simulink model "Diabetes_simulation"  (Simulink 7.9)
settings: Solver=ode4  SolverMode=SingleTasking  StartTime=0.0  StopTime=2880  FixedStep=parameters.passo_int  RelTol=1e-3
undefined symbols (not defined in the file or in its folder): boluses, meals, parameters
libraries: simulink x1

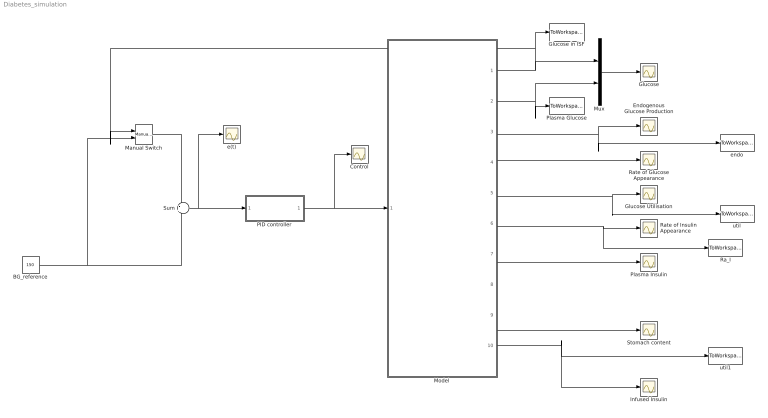
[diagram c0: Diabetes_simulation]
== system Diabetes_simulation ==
  BG_reference : Constant  Value=150
  Control : Scope
  Endogenous Glucose Production : Scope
  Glucose : Scope
  Glucose Utilisation : Scope
  Glucose in ISF : ToWorkspace  VariableName=G_ISF  SampleTime=-1
  Infused Insulin : Scope
  Manual Switch : simulink/Signal Routing/Manual Switch  sw=0  action=0  varsize=off
  Model : Subsystem
  Mux : Mux  Inputs=2
  PID controller : Subsystem
  Plasma Glucose : ToWorkspace  VariableName=G_P  SampleTime=-1
  Plasma Insulin : Scope
  Ra_I : ToWorkspace  VariableName=Ra_I  SampleTime=-1
  Rate of Glucose Appearance : Scope
  Rate of Insulin Appearance : Scope
  Stomach content : Scope
  Sum : Sum  Inputs=-+
  e(t) : Scope
  endo : ToWorkspace  VariableName=endo  SampleTime=-1
  util : ToWorkspace  VariableName=util  SampleTime=-1
  util1 : ToWorkspace  VariableName=infused  SampleTime=-1
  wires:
  Model/3(EGP) -> Endogenous Glucose Production/1, endo/1
  Model/4(Ra_g) -> Rate of Glucose Appearance/1
  Model/5(Util) -> Glucose Utilisation/1, util/1
  Model/6(Ra_I) -> Rate of Insulin Appearance/1, Ra_I/1
  Model/7(I_p) -> Plasma Insulin/1
  Model/9(q_tot) -> Stomach content/1
  Mux/1 -> Glucose/1
  Model/1("G_{ISF}") -> Mux/1, Glucose in ISF/1, Manual Switch/1
  Model/2(G_p) -> Mux/2, Plasma Glucose/1
  Sum/1 -> PID controller/1(In1), e(t)/1
  BG_reference/1 -> Sum/2, Manual Switch/2
  PID controller/1(Out1) -> Model/1(your controller), Control/1
  Model/10(Infused Insulin) -> util1/1, Infused Insulin/1
  Manual Switch/1 -> Sum/1

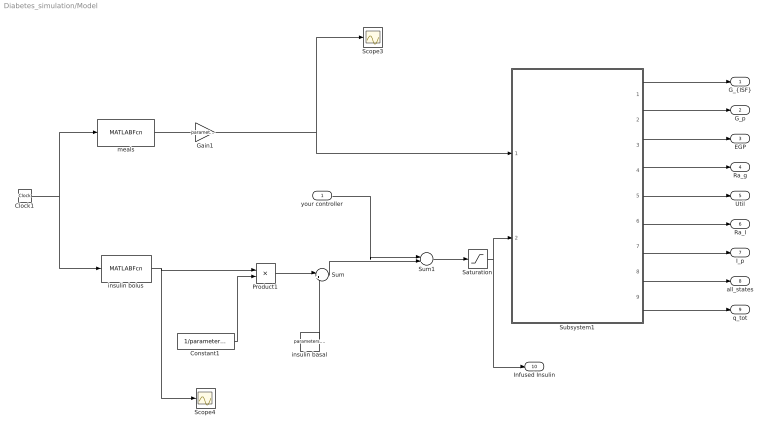
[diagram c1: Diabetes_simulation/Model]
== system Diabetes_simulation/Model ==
  your controller : Inport
  Clock1 : Clock
  Constant1 : Constant  Value=1/parameters.BW
  Gain1 : Gain  Gain=parameters.errpasti
  Product1 : Product
  Saturation : Saturate  UpperLimit=10000  LowerLimit=0
  Scope3 : Scope
  Scope4 : Scope
  Subsystem1 : Subsystem
  Sum : Sum  Inputs=|++
  Sum1 : Sum  Inputs=|++
  insulin basal : Constant  Value=parameters.u2ss
  insulin bolus : MATLABFcn  MATLABFcn=boluses(1,floor(u/parameters.passo_int)+1)  OutputDimensions=1  Output1D=off
  meals : MATLABFcn  MATLABFcn=meals(1,floor(u/parameters.passo_int)+1)  OutputDimensions=1  Output1D=off
  "G_{ISF}" : Outport
  G_p : Outport  Port=2
  EGP : Outport  Port=3
  Ra_g : Outport  Port=4
  Util : Outport  Port=5
  Ra_I : Outport  Port=6
  I_p : Outport  Port=7
  all_states : Outport  Port=8
  q_tot : Outport  Port=9
  Infused Insulin : Outport  Port=10
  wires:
  Subsystem1/1("G_{ISF}") -> "G_{ISF}"/1
  insulin basal/1 -> Sum/2
  meals/1 -> Gain1/1
  Product1/1 -> Sum/1
  Gain1/1 -> Subsystem1/1(In1), Scope3/1
  Constant1/1 -> Product1/2
  insulin bolus/1 -> Product1/1, Scope4/1
  Subsystem1/2(G_p) -> G_p/1
  Subsystem1/3(EGP) -> EGP/1
  Subsystem1/4(Ra) -> Ra_g/1
  Subsystem1/5(Util) -> Util/1
  Subsystem1/6(Ra_I) -> Ra_I/1
  Subsystem1/7(I_p) -> I_p/1
  Subsystem1/8(all_states) -> all_states/1
  Subsystem1/9(q_tot) -> q_tot/1
  Sum/1 -> Sum1/2
  Sum1/1 -> Saturation/1
  Clock1/1 -> meals/1, insulin bolus/1
  Saturation/1 -> Subsystem1/2(In2), Infused Insulin/1
  your controller/1 -> Sum1/1

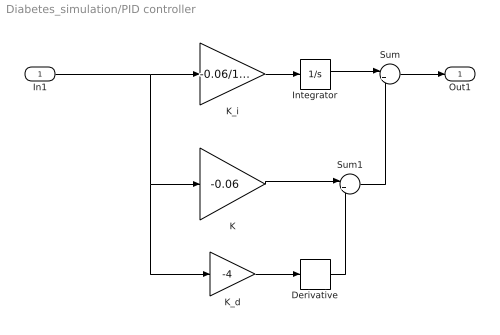
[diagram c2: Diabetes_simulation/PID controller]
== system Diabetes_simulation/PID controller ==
  In1 : Inport
  Derivative : Derivative
  Integrator : Integrator
  K : Gain  Gain=-0.06
  K_d : Gain  Gain=-4
  K_i : Gain  Gain=-0.06/1000
  Sum : Sum  Inputs=|++
  Sum1 : Sum  Inputs=|++
  Out1 : Outport
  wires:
  In1/1 -> K_i/1, K_d/1, K/1
  Sum/1 -> Out1/1
  Integrator/1 -> Sum/1
  K_i/1 -> Integrator/1
  K_d/1 -> Derivative/1
  Derivative/1 -> Sum1/2
  Sum1/1 -> Sum/2
  K/1 -> Sum1/1

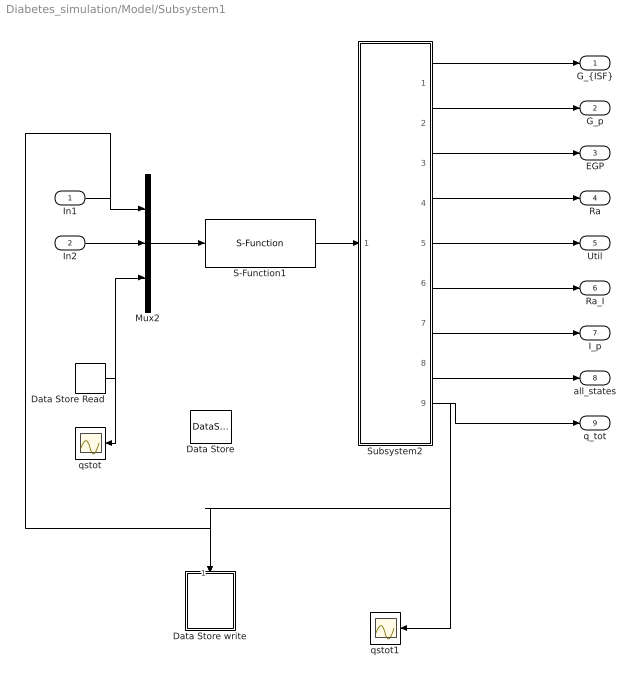
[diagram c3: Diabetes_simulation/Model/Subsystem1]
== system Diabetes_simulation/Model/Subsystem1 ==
  In1 : Inport
  In2 : Inport  Port=2
  Data Store : DataStoreMemory  DataStoreName=qstot
  Data Store Read : DataStoreRead  DataStoreName=qstot
  Data Store write : Subsystem  TreatAsAtomicUnit=on
  Mux2 : Mux  Inputs=3
  S-Function1 : S-Function  FunctionName=Padova_model  Parameters=parameters  EnableBusSupport=off
  Subsystem2 : Subsystem
  qstot : Scope
  qstot1 : Scope
  "G_{ISF}" : Outport
  G_p : Outport  Port=2
  EGP : Outport  Port=3
  Ra : Outport  Port=4
  Util : Outport  Port=5
  Ra_I : Outport  Port=6
  I_p : Outport  Port=7
  all_states : Outport  Port=8
  q_tot : Outport  Port=9
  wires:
  S-Function1/1 -> Subsystem2/1(In1)
  Subsystem2/1("G_{ISF}") -> "G_{ISF}"/1
  In2/1 -> Mux2/2
  Mux2/1 -> S-Function1/1
  In1/1 -> Mux2/1, Data Store write/Trigger
  Data Store Read/1 -> qstot/1, Mux2/3
  Subsystem2/9(q_tot) -> Data Store write/1(qsto), qstot1/1, q_tot/1
  Subsystem2/2(G_p) -> G_p/1
  Subsystem2/3(EGP) -> EGP/1
  Subsystem2/4(Ra) -> Ra/1
  Subsystem2/5(Util) -> Util/1
  Subsystem2/6(Ra_I) -> Ra_I/1
  Subsystem2/7(I_p) -> I_p/1
  Subsystem2/8(all_states) -> all_states/1

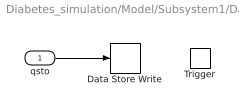
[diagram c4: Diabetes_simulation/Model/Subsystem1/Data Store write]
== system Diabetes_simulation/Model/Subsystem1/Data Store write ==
  qsto : Inport
  Trigger : TriggerPort
  Data Store Write : DataStoreWrite  DataStoreName=qstot
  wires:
  qsto/1 -> Data Store Write/1

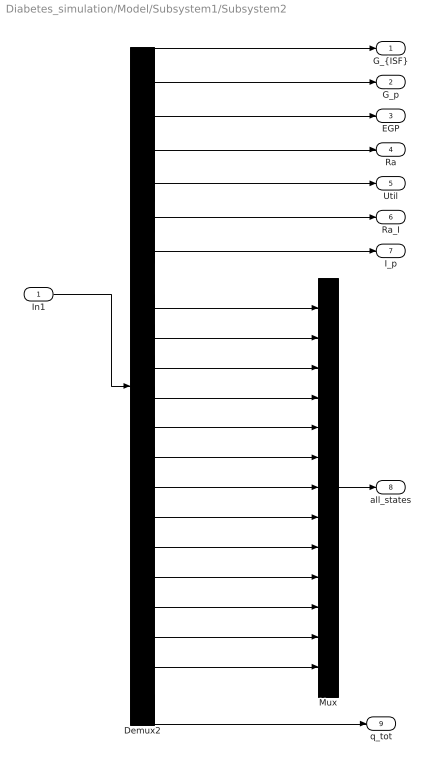
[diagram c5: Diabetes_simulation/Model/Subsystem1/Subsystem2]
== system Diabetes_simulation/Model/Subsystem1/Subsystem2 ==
  In1 : Inport
  Demux2 : Demux  Outputs=21
  Mux : Mux  Inputs=13
  "G_{ISF}" : Outport
  G_p : Outport  Port=2
  EGP : Outport  Port=3
  Ra : Outport  Port=4
  Util : Outport  Port=5
  Ra_I : Outport  Port=6
  I_p : Outport  Port=7
  all_states : Outport  Port=8
  q_tot : Outport  Port=9
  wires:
  In1/1 -> Demux2/1
  Demux2/1 -> "G_{ISF}"/1
  Demux2/2 -> G_p/1
  Demux2/3 -> EGP/1
  Demux2/4 -> Ra/1
  Demux2/5 -> Util/1
  Demux2/6 -> Ra_I/1
  Demux2/7 -> I_p/1
  Demux2/8 -> Mux/1
  Demux2/9 -> Mux/2
  Demux2/10 -> Mux/3
  Demux2/11 -> Mux/4
  Demux2/12 -> Mux/5
  Demux2/13 -> Mux/6
  Demux2/14 -> Mux/7
  Demux2/15 -> Mux/8
  Demux2/16 -> Mux/9
  Demux2/17 -> Mux/10
  Demux2/18 -> Mux/11
  Demux2/19 -> Mux/12
  Demux2/20 -> Mux/13
  Mux/1 -> all_states/1
  Demux2/21 -> q_tot/1
